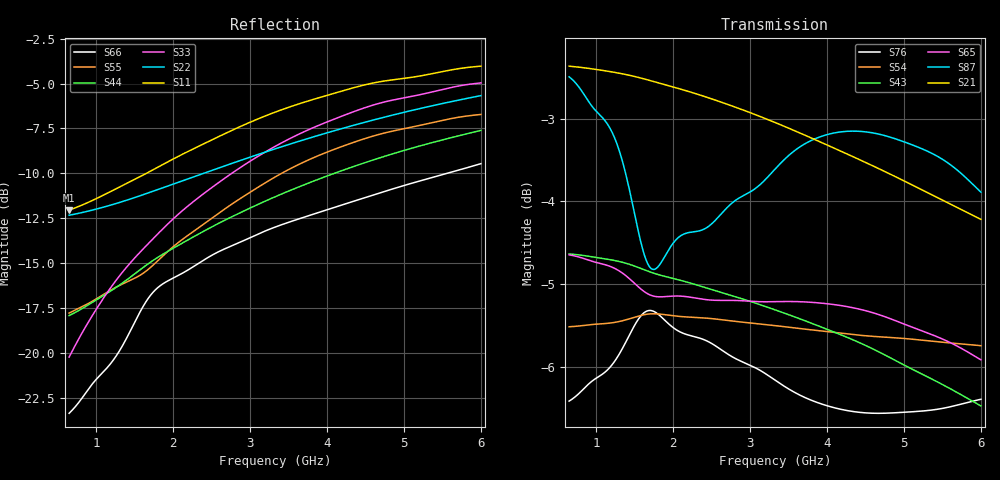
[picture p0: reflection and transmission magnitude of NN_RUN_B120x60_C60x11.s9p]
! IGNION VIRTUAL ANTENNA LIBRARY
! NN_RUN_B120x60_C60x11
! Virtual Antenna™ RUN mXTEND™: NN02-224 12.0 mm x 3.0 mm x 2.4 mm
! https://ignion.io/product/run-mxtend/
! Board: 120 mm x 60 mm
! Clearance Area: 60 mm x 11 mm
! Feeding line: L-shape; 11mm x 2mm and 5mm x 2mm
! Applications: Smartphone, Fleet management, IoT
! Frequency range 0.65GHz to 6GHz, step 10MHz
! Number of ports 9
! This product and its use is protected by at least one or more of the following patents and patent
! applications US 8,203,492 B2; US 8,237,615 B2; PCT/EP2013/064692; WO 2014/012842 A1; US 2019/190122 A1;
! US 62/072,671; and other domestic and international patents pending. Additional information about
! patents related to this product is available at https://ignion.io/files/Patent-list-NN.pdf, all
! rights reserved. Copyright, Ignion 2021.
! Need more help? Your platform is much different than these examples in the manual? Use our
! Fast Track service (https://ignion.io/fast-track/), for free, and get a personalized antenna design in
! just 24 hours.
! Touchstone port 1 = "Series Port"
! Touchstone port 2 = "Shunt Port"
! Touchstone port 3 = "Series Port"
! Touchstone port 4 = "Shunt Port"
! Touchstone port 5 = "Series Port"
! Touchstone port 6 = "Shunt Port"
! Touchstone port 7 = "Series Port"
! Touchstone port 8 = "Shunt Port"
! Touchstone port 9 = "Series Port"
! IE3D S-Parameters Output Version 2.0
# GHZ S MA R 50
! Nport = 9
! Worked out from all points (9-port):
!   536 points, 650 MHz to 6 GHz, reference 50 ohm
!   strongest paths, dB at 650 MHz, 1.99 GHz, 3.33 GHz, 4.67 GHz, 6 GHz:
!     S21: -2.4, -2.6, -3.0, -3.6, -4.2
!     S87: -2.5, -4.5, -3.6, -3.2, -3.9
!     S65: -4.6, -5.1, -5.2, -5.4, -5.9
!     S43: -4.6, -4.9, -5.3, -5.8, -6.5
!     S54: -5.5, -5.4, -5.5, -5.6, -5.7
!     S76: -6.4, -5.5, -6.2, -6.6, -6.4
!   lowest |S11| = -12.0 dB at 650 MHz (marker M1), VSWR 1.67, Z = 31.1 + j7.74 ohm
!   |S11| at or under -10 dB: start of sweep to 1.651 GHz
